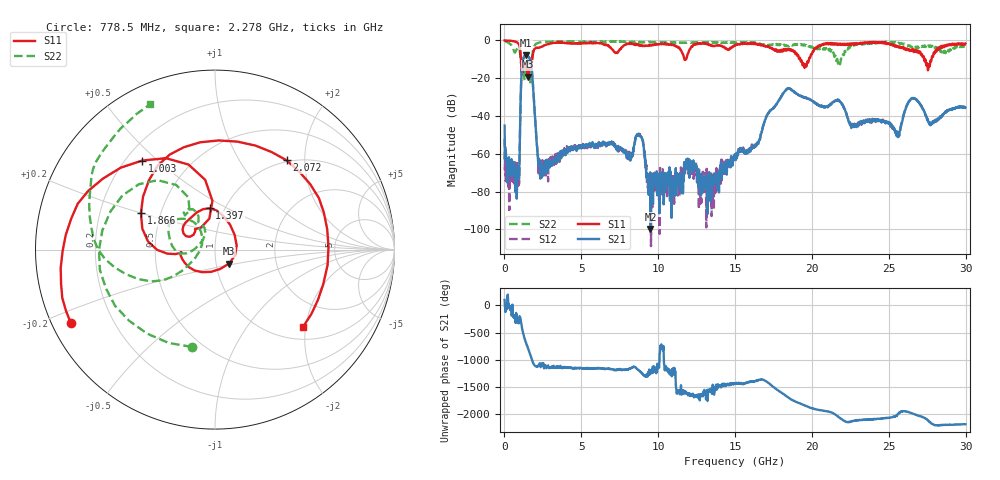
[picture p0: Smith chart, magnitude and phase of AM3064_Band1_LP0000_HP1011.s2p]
# Hz S DB R 50.0
!freq dBS11 angS11 dBS21 angS21 dBS12 angS12 dBS22 angS22
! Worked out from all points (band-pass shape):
!   1600 points, 10 MHz to 29.98 GHz, reference 50 ohm
!   highest |S21| = -7.85 dB at 1.397 GHz (marker M1); lowest = -99.8 dB at 9.494 GHz (marker M2)
!   |S21| within 3 dB of the highest: 1.191 GHz to 1.689 GHz (498.7 MHz wide, 34.6 % of centre)
!   lowest |S11| = -19.1 dB at 1.528 GHz (marker M3), VSWR 1.25, Z = 57.7 - j9.13 ohm
!   |S11| at or under -10 dB: 1.071 GHz to 1.807 GHz (736.7 MHz wide, 51.2 % of centre); 19.24 GHz to 19.8 GHz (562.6 MHz wide, 2.88 % of centre); 27.3 GHz to 27.78 GHz (481.5 MHz wide, 1.75 % of centre)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
!   |S22| runs from -22.3 to -0.2 dB; largest |S21 - S12| = 0.0052
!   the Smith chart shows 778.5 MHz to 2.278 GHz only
!   S11 on the Smith chart (normalised r, x): 778.5 MHz: 0.05, -0.24; 1.003 GHz: 0.27, +0.45; 1.397 GHz: 0.85, +0.41; 1.866 GHz: 0.39, +0.20; 2.072 GHz: 0.97, +1.63; 2.278 GHz: 1.29, -1.94
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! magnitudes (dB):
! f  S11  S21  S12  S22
! 10 MHz  0.0  -45.1  -52.0  -0.2
! 778.5 MHz  -0.9  -71.0  -77.1  -5.1
! 1.003 GHz  -3.9  -51.9  -51.0  -6.0
! 1.191 GHz  -16.8  -10.8  -10.8  -14.5
! 1.397 GHz  -12.7  -7.9  -7.9  -13.2
! 1.528 GHz  -19.1  -8.2  -8.2  -11.1
! 1.866 GHz  -6.7  -25.1  -25.0  -4.9
! 2.072 GHz  -3.9  -51.1  -50.9  -1.7
! 2.278 GHz  -3.7  -65.0  -63.6  -1.0
! 5.015 GHz  -1.5  -56.4  -57.2  -0.7
! 8.164 GHz  -1.8  -59.4  -61.9  -0.7
! 8.745 GHz  -2.7  -50.3  -50.0  -1.2
! 9.494 GHz  -2.5  -99.8  -73.8  -0.8
! 10 GHz  -2.0  -70.9  -73.7  -0.9
! 13.62 GHz  -2.9  -72.0  -89.9  -1.0
! 15 GHz  -2.8  -60.9  -60.3  -1.2
! 18.34 GHz  -5.4  -25.9  -25.8  -2.7
! 19.99 GHz  -7.3  -31.9  -31.8  -3.3
! 25 GHz  -1.5  -43.9  -43.9  -1.1
! 26.59 GHz  -5.4  -30.6  -30.7  -3.4
! 27.56 GHz  -15.3  -42.9  -43.8  -2.8
! 29.98 GHz  -1.6  -35.5  -35.4  -3.2
